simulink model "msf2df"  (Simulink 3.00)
settings: Solver=ode45  SolverMode=SingleTasking  StartTime=0.0  StopTime=300  MaxStep=10  RelTol=1e-5  AbsTol=1e-6
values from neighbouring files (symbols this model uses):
  d_through_p = get(MAIN_MENU(19),'Value')    [cback.m]    (also in imcmenu.m = 0)
  Disturb = Setpoint    [mimo_MSF1DF_sim.m]    (also in mimo_MSF2DF_sim.m)
  K = 1/kpd    [imc2pseucon.m]    (also in imc2pseudo.m)
  Satlb = temp1    [cback.m]    (also in imcmenu.m = str2num(satlbs))
  Satub = temp1    [cback.m]    (also in imcmenu.m = str2num(satubs))
  Setpoint = zeros(1,n)    [mimo_MSF1DF_sim.m]    (also in mimo_MSF2DF_sim.m)
undefined symbols (not defined in the file or in its folder): denFs, denMs, denPd, denPs, DrN, Ksp, Md, Mnt, NrD, numFs, numPd, numPs, Qdden, Qdnum
libraries: simulink3 x3, MIMO_lib x2

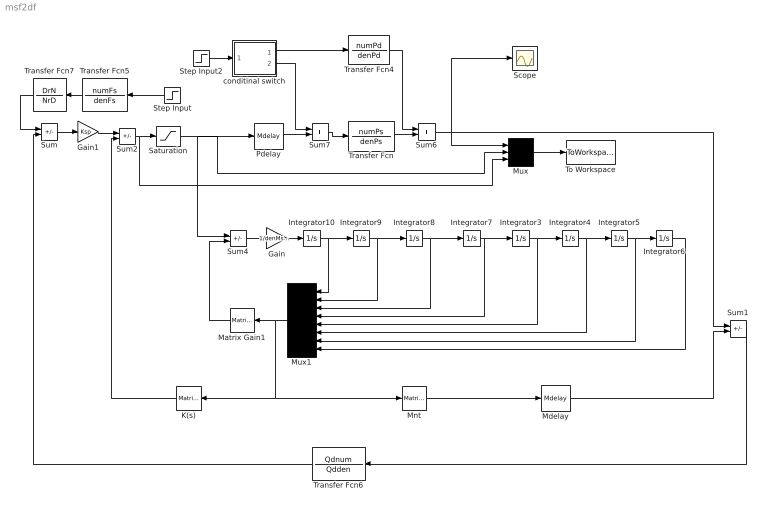
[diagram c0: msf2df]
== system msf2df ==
  Gain : Gain  Gain=1/denMs(1)  SaturateOnIntegerOverflow=on
  Gain1 : Gain  Gain=Ksp  SaturateOnIntegerOverflow=on
  Integrator{3..10} (8 alike) : Integrator  ExternalReset=none  InitialConditionSource=internal  InitialCondition=0  LimitOutput=off  UpperSaturationLimit=inf  LowerSaturationLimit=-inf  ShowSaturationPort=off  ShowStatePort=off  AbsoluteTolerance=auto
  K(s) : simulink3/Math/Matrix Gain  Orientation=left  K=K(2:9)
  Matrix Gain1 : simulink3/Math/Matrix Gain  Orientation=left  K=Md(2:9)
  Mdelay : MIMO_lib/Mdelay  Mdelay=Mdelay
  Mnt : simulink3/Math/Matrix Gain  K=Mnt
  Mux : Mux  Inputs=3
  Mux1 : Mux  Orientation=left  Inputs=8
  Pdelay : MIMO_lib/Mdelay  Mdelay=Pdelay
  Saturation : Saturate  UpperLimit=Satub  LowerLimit=Satlb
  Scope : Scope
  Step Input : Step  Orientation=left  Time=0  Before=0  After=Setpoint  SampleTime=0
  Step Input2 : Step  Time=0  Before=0  After=Disturb  SampleTime=0
  Sum{,1..2,4} (4 alike) : Sum  Inputs=+-  SaturateOnIntegerOverflow=on
  Sum6 : Sum  Inputs=++  SaturateOnIntegerOverflow=on
  Sum7 : Sum  Inputs=++  SaturateOnIntegerOverflow=on
  To Workspace : ToWorkspace  VariableName=simout  SampleTime=-1  SaveFormat=Matrix
  Transfer Fcn : TransferFcn  Numerator=numPs  Denominator=denPs
  Transfer Fcn4 : TransferFcn  Numerator=numPd  Denominator=denPd
  Transfer Fcn5 : TransferFcn  Orientation=left  Numerator=numFs  Denominator=denFs
  Transfer Fcn6 : TransferFcn  Orientation=left  Numerator=Qdnum  Denominator=Qdden
  Transfer Fcn7 : TransferFcn  Orientation=left  Numerator=DrN  Denominator=NrD
  conditinal switch : Subsystem  Description=pass input signal through out1 if condition is true.
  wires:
  Sum/1 -> Gain1/1
  Gain1/1 -> Sum2/1
  Mdelay/1 -> Sum1/2
  Sum1/1 -> Transfer Fcn6/1
  Sum2/1 -> Saturation/1, Mux/3
  Gain/1 -> Integrator10/1
  Sum4/1 -> Gain/1
  Transfer Fcn7/1 -> Sum/1
  Transfer Fcn5/1 -> Transfer Fcn7/1
  Step Input/1 -> Transfer Fcn5/1
  Integrator10/1 -> Integrator9/1, Mux1/1
  Integrator9/1 -> Integrator8/1, Mux1/2
  Integrator8/1 -> Integrator7/1, Mux1/3
  Integrator7/1 -> Integrator3/1, Mux1/4
  Integrator3/1 -> Integrator4/1, Mux1/5
  Integrator4/1 -> Integrator5/1, Mux1/6
  Integrator5/1 -> Integrator6/1, Mux1/7
  Integrator6/1 -> Mux1/8
  Sum6/1 -> Mux/1, Sum1/1, Scope/1
  Matrix Gain1/1 -> Sum4/2
  Mux1/1 -> Matrix Gain1/1, K(s)/1, Mnt/1
  K(s)/1 -> Sum2/2
  Mnt/1 -> Mdelay/1
  Transfer Fcn6/1 -> Sum/2
  Transfer Fcn/1 -> Sum6/2
  Sum7/1 -> Transfer Fcn/1
  Pdelay/1 -> Sum7/2
  Saturation/1 -> Sum4/1, Mux/2, Pdelay/1
  Transfer Fcn4/1 -> Sum6/1
  conditinal switch/2(Out1) -> Sum7/1
  conditinal switch/1(Out2) -> Transfer Fcn4/1
  Step Input2/1 -> conditinal switch/1(In)
  Mux/1 -> To Workspace/1

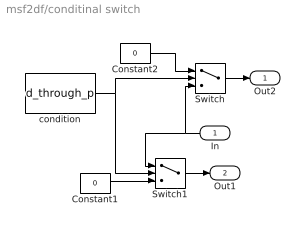
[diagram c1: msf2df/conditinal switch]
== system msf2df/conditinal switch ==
  In : Inport  Orientation=left  Port=1  PortWidth=-1  SampleTime=-1  DataType=auto
  Constant1 : Constant  Value=0
  Constant2 : Constant  Value=0
  Switch : Switch  Threshold=1
  Switch1 : Switch  Threshold=1
  condition : Constant  Value=d_through_p
  Out2 : Outport  Port=1  InitialOutput=0
  Out1 : Outport  Port=2  InitialOutput=0
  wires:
  In/1 -> Switch/3, Switch1/1
  condition/1 -> Switch1/2, Switch/2
  Constant1/1 -> Switch1/3
  Constant2/1 -> Switch/1
  Switch/1 -> Out2/1
  Switch1/1 -> Out1/1
